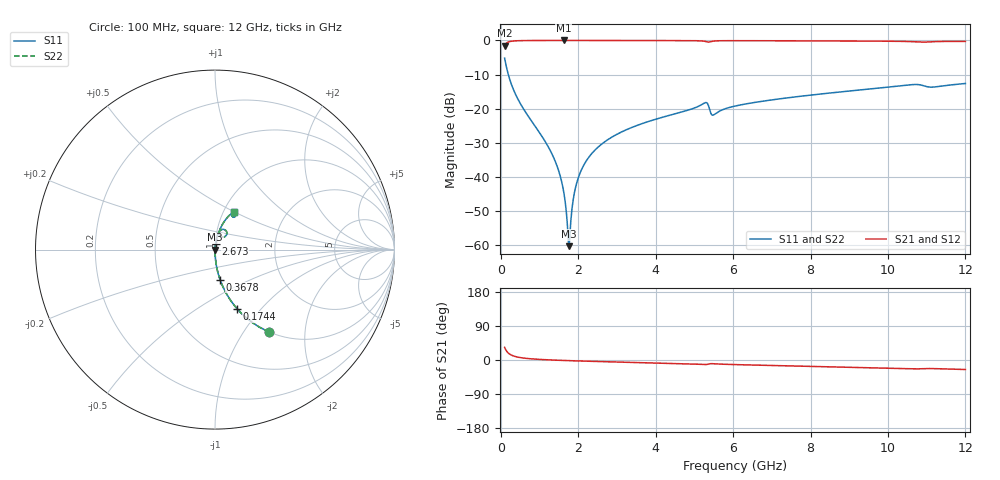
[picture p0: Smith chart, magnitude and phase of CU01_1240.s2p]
! S-parameter model data by Modelithics Inc. support@modelithics.com 813-866-6335 Tampa FL USA
! S-Parameter data specifications:
! Substrate: 20-mil Rogers, substrate thickness, H=0.508mm, Dielectric constant, Er=3.75
! PCB Mounting Pad Footprint: Pad width, PadW=0.35mm , Pad length, PadL=0.30mm , Pad gap, PadG (edge-to-edge)=0.25mm , Reference planes=0.85mm apart
! Created Tue May  8 14:01:25 2018
# hz S ma R 50
! 2 Port Network Data from SP1.SP block
! freq  magS11  angS11  magS21  angS21  magS12  angS12  magS22  angS22
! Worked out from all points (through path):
!   801 points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, 100 MHz to 12 GHz, reference 50 ohm
!   highest |S21| = -0.01 dB at 1.632 GHz (marker M1); lowest = -1.6 dB at 100 MHz (marker M2)
!   group delay of S21, straight-line fit = 7.21 ps
!   lowest |S11| = -60.2 dB at 1.766 GHz (marker M3), VSWR 1.00, Z = 50.1 + j0.0167 ohm
!   |S11| at or under -10 dB: 196.1 MHz to end of sweep
!   |S22| runs from -60.2 to -5.2 dB; largest |S21 - S12| = 0
!   S11 on the Smith chart (normalised r, x): 100 MHz: 1.00, -1.32; 174.4 MHz: 1.00, -0.75; 367.8 MHz: 1.00, -0.34; 2.673 GHz: 1.01, +0.06; 12 GHz: 1.11, +0.50
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1e8  0.5504 -56.7  0.8346 33.3  0.8346 33.3  0.5504 -56.7
1.74375e8  0.3516 -69.5  0.9358 20.4  0.9358 20.4  0.3516 -69.5
3.6775e8  0.1695 -80.4  0.9851 9.4  0.9851 9.4  0.1695 -80.4
1.31975e9  0.02202 -87.8  0.9989 -0.0  0.9989 -0.0  0.02202 -87.8
1.513125e9  0.01151 -86.4  0.999 -0.8  0.999 -0.8  0.01151 -86.4
1.632125e9  0.005816 -82.1  0.999 -1.2  0.999 -1.2  0.005816 -82.1
1.721375e9  0.001972 -63.0  0.999 -1.6  0.999 -1.6  0.001972 -63.0
1.766e9  0.0009751 9.8  0.999 -1.7  0.999 -1.7  0.0009751 9.8
1.810625e9  0.002289 63.1  0.999 -1.9  0.999 -1.9  0.002289 63.1
1.870125e9  0.004618 75.7  0.999 -2.1  0.999 -2.1  0.004618 75.7
1.91475e9  0.006372 78.8  0.999 -2.2  0.999 -2.2  0.006372 78.8
2.09325e9  0.01311 82.7  0.9988 -2.8  0.9988 -2.8  0.01311 82.7
2.33125e9  0.02145 83.6  0.9986 -3.5  0.9986 -3.5  0.02145 83.6
2.673375e9  0.03247 83.5  0.9983 -4.4  0.9983 -4.4  0.03247 83.5
3.2535e9  0.04956 82.5  0.9974 -6.0  0.9974 -6.0  0.04956 82.5
4.071625e9  0.07219 80.7  0.9958 -8.1  0.9958 -8.1  0.07219 80.7
5.2765e9  0.1225 66.8  0.9689 -12.0  0.9689 -12.0  0.1225 66.8
5.48475e9  0.08074 65.2  0.9759 -9.8  0.9759 -9.8  0.08074 65.2
6.05e9  0.1095 76.4  0.9911 -12.1  0.9911 -12.1  0.1095 76.4
8.04325e9  0.1594 72.3  0.9849 -16.9  0.9849 -16.9  0.1594 72.3
1.002162e10  0.2074 67.2  0.974 -21.6  0.974 -21.6  0.2074 67.2
1.2e10  0.2342 63.8  0.9674 -25.1  0.9674 -25.1  0.2342 63.8
